DATA_BLOCK "Demo4"
VERSION : 0.1


  STRUCT
   str1 : STRING  [254 ] := '135 ACEGJLNP';	//write $$ to insert one single $; write $R to insert <CR> (0d hex)
  END_STRUCT ;
BEGIN
   str1 := '135 ACEGJLNP';
END_DATA_BLOCK

